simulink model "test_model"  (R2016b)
settings: Solver=VariableStepAuto  StartTime=0.0  StopTime=runtime  RelTol=1e-3
InitFcn:
  | clear mex
  | delete test_model_sfun.mexw64
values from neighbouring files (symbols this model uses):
  g = 9.81    [modelParameters.m]
  height_controlled_o = (((Rm*If        + (((omega0_o * 2 * Rm * Kv * Kq      * Kd + 1)^2) - 1)/(4* Rm*Kv^2*Kq      * Kd))/Vb)*(Pmax - Pmin) + Pmin)    [modelParameters.m]
  If = 0.3836    [modelParameters.m]
  Jreq = 4.2012e-05    [modelParameters.m]
  Jxx = 0.0130    (= 0.013)    [modelParameters.m]
  Jyy = 0.0140    (= 0.014)    [modelParameters.m]
  Jzz = 0.0285    [modelParameters.m]
  Kd = 1.4852e-07    [modelParameters.m]
  Ki_mahony = 0.001    [modelParameters.m]
  Kp_mahony = 0.4    [modelParameters.m]
  Kq = 96.3422    [modelParameters.m]
  Kt = 1.2007e-05    [modelParameters.m]
  Kv = 96.3422    [modelParameters.m]
  m = 1.216    [modelParameters.m]
  omega0_o = sqrt((m*g)/(4*Kt))    [modelParameters.m]
  omega1_o = sqrt((m*g)/(4*Kt))    [modelParameters.m]
  omega2_o = sqrt((m*g)/(4*Kt))    [modelParameters.m]
  omega3_o = sqrt((m*g)/(4*Kt))    [modelParameters.m]
  pitch_o = 0    [modelParameters.m]
  pitchrate_o = 0    [modelParameters.m]
  Pmax = 1    [modelParameters.m]
  Pmin = 0    [modelParameters.m]
  r_oc = [0; 0; 0]    [modelParameters.m]
  rhx = 0.16    [modelParameters.m]
  rhy = 0.16    [modelParameters.m]
  rhz = 0.03    [modelParameters.m]
  Rm = 0.235    [modelParameters.m]
  roll_o = 0    [modelParameters.m]
  rollrate_o = 0    [modelParameters.m]
  Tc = 0.04    [modelParameters.m]
  Tq = 0.005    [modelParameters.m]
  Vb = 11.4    [modelParameters.m]
  x_controlled_o = 0    [modelParameters.m]
  x_o = 0    [modelParameters.m]
  x_vel_o = 0    [modelParameters.m]
  y_controlled_o = 0    [modelParameters.m]
  y_o = 0    [modelParameters.m]
  y_vel_o = 0    [modelParameters.m]
  yaw_controlled_o = 0    [modelParameters.m]
  yaw_o = 0    [modelParameters.m]
  yawrate_o = 0    [modelParameters.m]
  z_o = 0    [modelParameters.m]
  z_vel_o = 0    [modelParameters.m]
undefined symbols (not defined in the file or in its folder): a, Ki, Kp, Ts
libraries: simulink x38, dsparch4 x3, vrlib x2
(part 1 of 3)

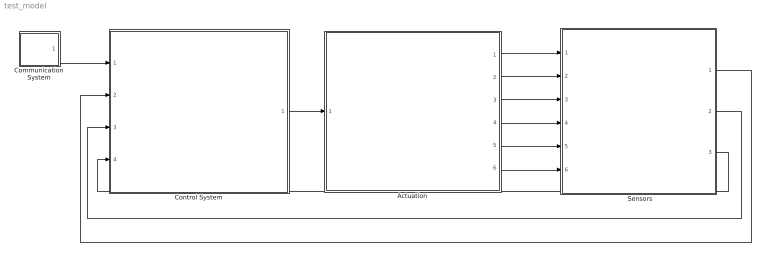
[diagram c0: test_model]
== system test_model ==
  "     Sensors   " : Subsystem
  Actuation : Subsystem
  Communication System : Subsystem
  Control System : Subsystem
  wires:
  Control System/1(P) -> Actuation/1(P)
  Communication System/1(setpoints) -> Control System/1(setpoints)
  Actuation/1(B_omega) -> "     Sensors   "/1(B_Omega)
  Actuation/2(euler_angles) -> "     Sensors   "/2(euler_angles)
  Actuation/3(B_vo) -> "     Sensors   "/3(B_vo)
  Actuation/4(E_ro) -> "     Sensors   "/4(E_ro)
  Actuation/5(B_vo_dot) -> "     Sensors   "/5(B_vo_dot)
  Actuation/6(B_g) -> "     Sensors   "/6(B_g)
  "     Sensors   "/3(current_position) -> Control System/4(current_position)
  "     Sensors   "/2(euler_rates) -> Control System/3(euler_rates)
  "     Sensors   "/1(euler_angles_filtered) -> Control System/2(euler_angles_filtered)

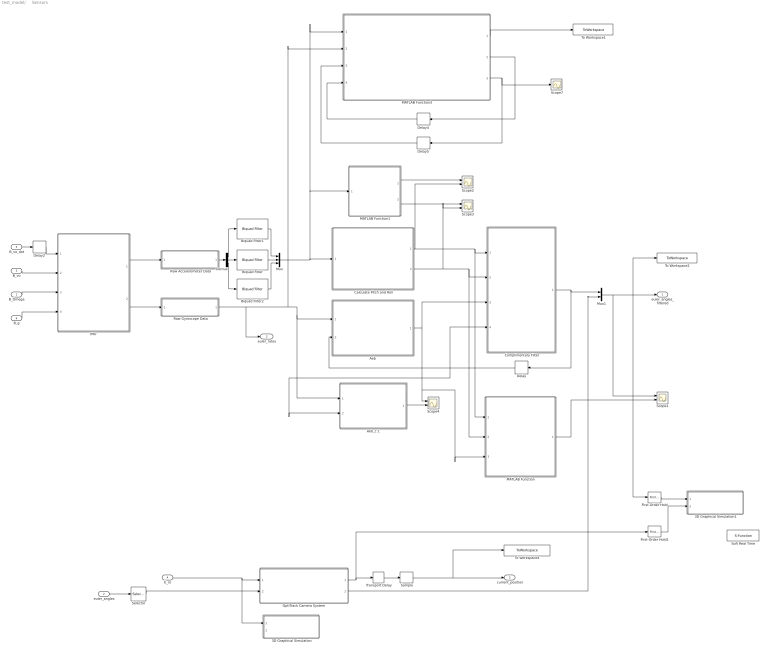
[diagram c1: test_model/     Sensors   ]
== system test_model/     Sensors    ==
  B_Omega : Inport
  euler_angles : Inport  Port=2
  B_vo : Inport  Port=3
  E_ro : Inport  Port=4
  B_vo_dot : Inport  Port=5
  B_g : Inport  Port=6
  3D Graphical Simulation : Subsystem  Commented=on
  3D Graphical Simulation1 : Subsystem  Commented=on
  "Aeb " : MATLAB Function  TreatAsAtomicUnit=on
  Aeb_c 1 : MATLAB Function  TreatAsAtomicUnit=on
  Biquad Filter : dsparch4/Biquad Filter  IIRFiltStruct=Direct form II  CoeffSource=Specify via dialog  BiQuadCoeffs=SOS_Matrix  a0Flag=Warning  IC=0  ICnum=0  ICden=0  InputProcessing=Columns as channels (frame based)  denAccumFracLength=30  denProdOutputFracLength=30  secondMemoryFracLength=15  roundingMode=Floor  overflowMode=off  ScaleValues=1  optimizeScaleValues=on  ScaleValueMode=Specify via input port (g)  scaleValueFracLength=14  FilterSource=Specify via dialog  FilterObject=BQF
  Biquad Filter1 : dsparch4/Biquad Filter  IIRFiltStruct=Direct form II  CoeffSource=Specify via dialog  BiQuadCoeffs=SOS_Matrix  a0Flag=Warning  IC=0  ICnum=0  ICden=0  InputProcessing=Columns as channels (frame based)  denAccumFracLength=30  denProdOutputFracLength=30  secondMemoryFracLength=15  roundingMode=Floor  overflowMode=off  ScaleValues=1  optimizeScaleValues=on  ScaleValueMode=Specify via input port (g)  scaleValueFracLength=14  FilterSource=Specify via dialog  FilterObject=BQF
  Biquad Filter2 : dsparch4/Biquad Filter  IIRFiltStruct=Direct form II  CoeffSource=Specify via dialog  BiQuadCoeffs=SOS_Matrix  a0Flag=Warning  IC=0  ICnum=0  ICden=0  InputProcessing=Columns as channels (frame based)  denAccumFracLength=30  denProdOutputFracLength=30  secondMemoryFracLength=15  roundingMode=Floor  overflowMode=off  ScaleValues=1  optimizeScaleValues=on  ScaleValueMode=Specify via input port (g)  scaleValueFracLength=14  FilterSource=Specify via dialog  FilterObject=BQF
  Calculate Pitch and Roll : MATLAB Function  TreatAsAtomicUnit=on
  Complimentary Filter : MATLAB Function  TreatAsAtomicUnit=on
  Delay : Delay  DelayLength=1  InitialCondition=0
  Delay2 : Delay  DelayLength=1  InitialCondition=0  SampleTime=Tq
  Delay4 : Delay  DelayLength=1  InitialCondition=0  SampleTime=Tq
  Delay5 : Delay  DelayLength=1  InitialCondition=[1, 0, 0, 0]  SampleTime=Tq
  Demux : Demux  Outputs=3
  First-Order Hold : simulink/Discrete/First-Order Hold  DisableCoverage=on  Ts=5e-3
  First-Order Hold1 : simulink/Discrete/First-Order Hold  DisableCoverage=on  Ts=5e-3
  "IMU " : Subsystem
  MATLAB Function : MATLAB Function  TreatAsAtomicUnit=on
  MATLAB Function1 : MATLAB Function  TreatAsAtomicUnit=on
  MATLAB Function3 : MATLAB Function  TreatAsAtomicUnit=on
  Mux : Mux  Inputs=3
  Mux1 : Mux  Inputs=2
  "OptiTrack Camera System " : Subsystem
  Raw Accelerometer Data : Subsystem  Variant=on
  Raw Gyroscope Data : Subsystem  Variant=on
  Sample : ZeroOrderHold  SampleTime=Tc
  Scope{1..4} (4 alike) : Scope  NumInputPorts=2
  Scope7 : Scope
  Selector : Selector  InputPortWidth=3  IndexOptions=Index vector (dialog)  Indices=[3]  OutputSizes=1
  Soft Real Time : S-Function  Commented=on  FunctionName=sfun_time  Parameters=x  SFunctionDeploymentMode=off  EnableBusSupport=off
  To Workspace1 : ToWorkspace  VariableName=mahony_reading  SaveFormat=Structure With Time  SampleTime=Tq
  To Workspace2 : ToWorkspace  VariableName=angle_IMU_reading  SaveFormat=Structure With Time  SampleTime=Tq
  To Workspace4 : ToWorkspace  VariableName=position_model  SaveFormat=Structure With Time  SampleTime=Tc
  Transport Delay : TransportDelay  DelayTime=6e-3
  euler_angles_filtered : Outport
  euler_rates : Outport  Port=2
  current_position : Outport  Port=3
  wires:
  "IMU "/1(accelerometer) -> Raw Accelerometer Data/1(raw_accel_model)
  "IMU "/2(gyroscope) -> Raw Gyroscope Data/1(raw_gyro_model)
  B_vo/1 -> "IMU "/2(B_vo)
  B_Omega/1 -> "IMU "/3(B_Omega)
  B_g/1 -> "IMU "/4(B_g)
  Calculate Pitch and Roll/2(accel_roll) -> Scope3/2, MATLAB Function/2(accel_roll), Complimentary Filter/2(accel_roll)
  Calculate Pitch and Roll/1(accel_pitch) -> MATLAB Function/1(accel_pitch), Complimentary Filter/1(accel_pitch), Scope2/2
  First-Order Hold/1 -> 3D Graphical Simulation1/1("Euler Angles ")
  E_ro/1 -> 3D Graphical Simulation/1(Displacement), "OptiTrack Camera System "/1(E_ro)
  First-Order Hold1/1 -> 3D Graphical Simulation1/2(Displacement)
  B_vo_dot/1 -> Delay2/1
  Delay2/1 -> "IMU "/1(B_vo_dot)
  "OptiTrack Camera System "/1(E_ro_camera) -> Transport Delay/1, First-Order Hold1/1
  Transport Delay/1 -> Sample/1
  Sample/1 -> To Workspace4/1, current_position/1
  Raw Gyroscope Data/1(raw_gyro) -> Aeb_c 1/1(gyro_reading), "Aeb "/1(gyro_reading), MATLAB Function3/2(gyroReadings), euler_rates/1
  Delay/1 -> Complimentary Filter/4(prev_euler_angles), Aeb_c 1/2(euler_angles_filtered), "Aeb "/2(euler_angles_filtered)
  Aeb_c 1/1(euler_rates_IMU) -> Scope4/2
  MATLAB Function1/1(accel_pitch) -> Scope2/1
  MATLAB Function1/2(accel_roll) -> Scope3/1
  "OptiTrack Camera System "/2(yaw_camera) -> Mux1/2
  MATLAB Function3/1(eulerAngles) -> To Workspace1/1
  MATLAB Function3/2(integralFeedback) -> Delay4/1
  Delay4/1 -> MATLAB Function3/4(integralFeedback_prev)
  MATLAB Function3/3(quaternions) -> Scope7/1, Delay5/1
  Delay5/1 -> MATLAB Function3/3(quaternions_prev)
  "Aeb "/1(euler_rates_IMU) -> MATLAB Function/3(euler_rates_gyro), Scope4/1, Complimentary Filter/3(euler_rates_gyro)
  Raw Accelerometer Data/1(raw_accel) -> Demux/1
  Demux/2 -> Biquad Filter/1
  Demux/1 -> Biquad Filter1/1
  Demux/3 -> Biquad Filter2/1
  Biquad Filter/1 -> Mux/2
  Biquad Filter1/1 -> Mux/1
  Biquad Filter2/1 -> Mux/3
  Mux/1 -> Calculate Pitch and Roll/1(accel_reading), MATLAB Function1/1(accel_reading), MATLAB Function3/1(accelReadings)
  Complimentary Filter/1(euler_angles_IMU) -> Mux1/1, Delay/1
  euler_angles/1 -> Selector/1
  Selector/1 -> "OptiTrack Camera System "/2(yaw)
  MATLAB Function/1(euler_angles_IMU) -> Scope1/2
  Mux1/1 -> Scope1/1, To Workspace2/1, First-Order Hold/1, euler_angles_filtered/1

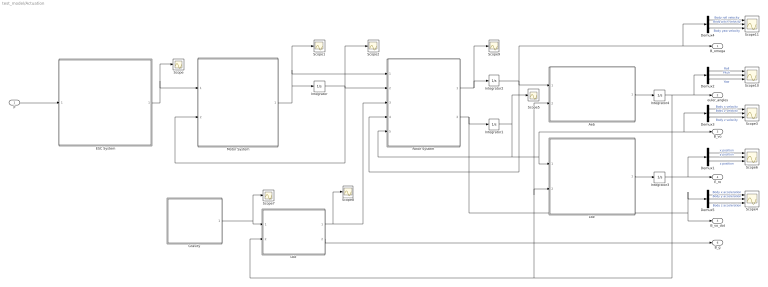
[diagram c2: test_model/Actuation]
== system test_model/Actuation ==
  P : Inport
  "Aeb " : MATLAB Function  TreatAsAtomicUnit=on
  Demux{1..5} (5 alike) : Demux  Outputs=3
  ESC System : MATLAB Function  TreatAsAtomicUnit=on
  "Gravity " : MATLAB Function  TreatAsAtomicUnit=on
  Integrator : Integrator  InitialCondition=[omega0_o, omega1_o, omega2_o, omega3_o]
  Integrator1 : Integrator  InitialCondition=[x_vel_o; y_vel_o; z_vel_o]
  Integrator2 : Integrator  InitialCondition=[rollrate_o; pitchrate_o; yawrate_o]
  Integrator3 : Integrator  InitialCondition=[x_o; y_o; z_o]
  Integrator4 : Integrator  InitialCondition=[roll_o; pitch_o; yaw_o]  ContinuousStateAttributes=['phi' 'theta' 'psi']
  "Lbe " : MATLAB Function  TreatAsAtomicUnit=on
  "Lbe " : MATLAB Function  TreatAsAtomicUnit=on
  Motor System : MATLAB Function  TreatAsAtomicUnit=on
  "Rotor System " : MATLAB Function  TreatAsAtomicUnit=on
  Scope{,1..2,5,7..9} (7 alike) : Scope
  Scope{3..4,6,10..11} (5 alike) : Scope  NumInputPorts=3
  B_omega : Outport
  euler_angles : Outport  Port=2
  B_vo : Outport  Port=3
  E_ro : Outport  Port=4
  B_vo_dot : Outport  Port=5
  B_g : Outport  Port=6
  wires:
  ESC System/1(Vb_eff) -> Scope/1, Motor System/1(Vb_eff)
  Motor System/1(w_dot) -> Integrator/1, Scope1/1, "Rotor System "/1(w_dot)
  "Rotor System "/1(B_omega_dot) -> Scope9/1, Integrator2/1
  Integrator2/1 -> "Rotor System "/4(B_omega), B_omega/1, Demux4/1, "Aeb "/1(B_omega)
  "Aeb "/1(euler_rates) -> Integrator4/1
  "Lbe "/1(E_ro) -> Integrator3/1
  Integrator3/1 -> Demux1/1, E_ro/1
  "Lbe "/1(B_Fg) -> Scope8/1, "Rotor System "/3(B_Fg)
  "Lbe "/2(B_g) -> B_g/1
  Demux1/2 -> Scope6/2  "y position"
  Demux1/1 -> Scope6/1  "x position"
  Demux1/3 -> Scope6/3  "z position"
  Demux2/2 -> Scope10/2  "Pitch"
  Demux2/1 -> Scope10/1  "Roll"
  Demux2/3 -> Scope10/3  "Yaw"
  Demux4/2 -> Scope11/2  "Body pitch velocity"
  Demux4/1 -> Scope11/1  "Body roll velocity"
  Demux4/3 -> Scope11/3  "Body yaw velocity"
  Demux3/2 -> Scope3/2  "Body y velocity"
  Demux3/1 -> Scope3/1  "Body x velocity"
  Demux3/3 -> Scope3/3  "Body z velocity"
  Demux5/2 -> Scope4/2  "Body y acceleration"
  Demux5/1 -> Scope4/1  "Body x acceleration"
  Demux5/3 -> Scope4/3  "Body z acceleration"
  Integrator1/1 -> Scope5/1, "Rotor System "/5(B_vo), "Lbe "/1(B_vo), Demux3/1, B_vo/1
  "Rotor System "/2(B_vo_dot) -> Demux5/1, B_vo_dot/1, Integrator1/1
  Integrator4/1 -> euler_angles/1, Demux2/1, "Lbe "/2(euler_angles), "Aeb "/2(euler_angles), "Lbe "/2(euler_angles)
  P/1 -> ESC System/1(P)
  "Gravity "/1(E_Fg) -> Scope7/1, "Lbe "/1(E_Fg)
  Integrator/1 -> Motor System/2(w), "Rotor System "/2(w), Scope2/1

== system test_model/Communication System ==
  Step : Step  Before=[0; 0; 0; 0]  After=[0; 1; 0; 0]  SampleTime=Tq
  setpoints : Outport
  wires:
  Step/1 -> setpoints/1

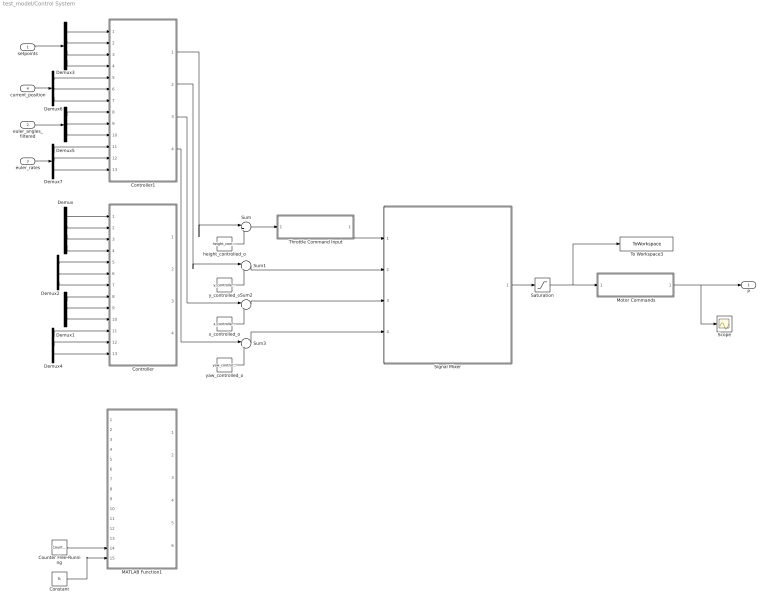
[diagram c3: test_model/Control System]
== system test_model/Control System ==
  setpoints : Inport
  euler_angles_filtered : Inport  Port=2
  euler_rates : Inport  Port=3
  current_position : Inport  Port=4
  Constant : Constant  Value=Tc  SampleTime=Tc
  Controller : Subsystem  Commented=on
  Controller1 : Subsystem
  Counter Free-Running : simulink/Sources/Counter Free-Running  NumBits=32  tsamp=Tc
  Demux : Demux
  Demux{1..2,4..7} (6 alike) : Demux  Outputs=3
  Demux3 : Demux
  MATLAB Function1 : MATLAB Function  Commented=on  TreatAsAtomicUnit=on  SystemSampleTime=Tq
  Motor Commands : Subsystem  Variant=on
  Saturation : Saturate  UpperLimit=Pmax*ones(4,1)  LowerLimit=Pmin*ones(4,1)
  Scope : Scope
  Signal Mixer : MATLAB Function  TreatAsAtomicUnit=on
  Sum{,1..3} (4 alike) : Sum  Inputs=|++
  Throttle Command Input : Subsystem  Variant=on
  To Workspace3 : ToWorkspace  VariableName=motorCommands  SaveFormat=Structure With Time  SampleTime=Tq
  height_controlled_o : Constant  Value=height_controlled_o  SampleTime=Tc
  x_controlled_o : Constant  Value=x_controlled_o
  y_controlled_o : Constant  Value=y_controlled_o
  yaw_controlled_o : Constant  Value=yaw_controlled_o
  P : Outport
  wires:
  Demux/1 -> Controller/1(x_setpoint)
  Demux/2 -> Controller/2(y_setpoint)
  Demux/3 -> Controller/3(z_setpoint)
  Demux2/1 -> Controller/5(x_position)
  Demux2/2 -> Controller/6(y_position)
  Demux2/3 -> Controller/7(z_position)
  y_controlled_o/1 -> Sum1/2
  x_controlled_o/1 -> Sum2/2
  yaw_controlled_o/1 -> Sum3/2
  Signal Mixer/1(P) -> Saturation/1
  Demux1/1 -> Controller/8(roll)
  Demux1/2 -> Controller/9(pitch)
  Demux4/1 -> Controller/11(roll_rate)
  Demux4/2 -> Controller/12(pitch_rate)
  Demux4/3 -> Controller/13(yaw_rate)
  Demux/4 -> Controller/4(yaw_setpoint)
  Demux1/3 -> Controller/10(yaw)
  Counter Free-Running/1 -> MATLAB Function1/14(vrpn_id)
  Constant/1 -> MATLAB Function1/15(Tc)
  Sum1/1 -> Signal Mixer/2(y_controlled)
  Sum2/1 -> Signal Mixer/3(x_controlled)
  Sum3/1 -> Signal Mixer/4(yaw_controlled)
  Throttle Command Input/1(z_command) -> Signal Mixer/1(height_controlled)
  height_controlled_o/1 -> Sum/2
  Motor Commands/1(z_command) -> P/1, Scope/1
  Sum/1 -> Throttle Command Input/1(z_command_model)
  Saturation/1 -> To Workspace3/1, Motor Commands/1(z_command_model)
  setpoints/1 -> Demux3/1
  current_position/1 -> Demux6/1
  euler_angles_filtered/1 -> Demux5/1
  euler_rates/1 -> Demux7/1
  Demux3/1 -> Controller1/1(x_setpoint)
  Demux3/2 -> Controller1/2(y_setpoint)
  Demux3/3 -> Controller1/3(z_setpoint)
  Demux3/4 -> Controller1/4(yaw_setpoint)
  Demux6/1 -> Controller1/5(x_position)
  Demux6/2 -> Controller1/6(y_position)
  Demux6/3 -> Controller1/7(z_position)
  Demux5/1 -> Controller1/8(roll)
  Demux5/2 -> Controller1/9(pitch)
  Demux5/3 -> Controller1/10(yaw)
  Demux7/1 -> Controller1/11(roll_rate)
  Demux7/2 -> Controller1/12(pitch_rate)
  Demux7/3 -> Controller1/13(yaw_rate)
  Controller1/4(yaw_controlled) -> Sum3/1
  Controller1/3(x_controlled) -> Sum2/1
  Controller1/2(y_controlled) -> Sum1/1
  Controller1/1(height_controlled) -> Sum/1

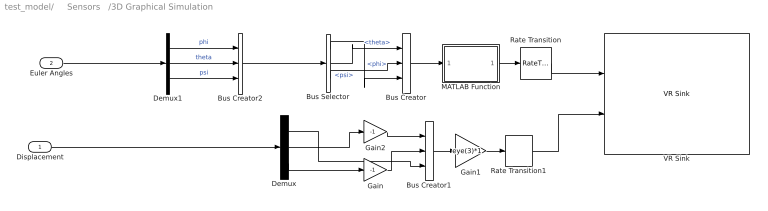
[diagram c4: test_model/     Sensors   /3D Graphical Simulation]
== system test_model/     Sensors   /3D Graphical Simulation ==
  Displacement : Inport
  Euler Angles : Inport  Port=2
  Bus Creator : BusCreator  Inputs=3
  Bus Creator1 : BusCreator  Inputs=3
  Bus Creator2 : BusCreator  Inputs=3
  Bus Selector : BusSelector  OutputSignals=phi,theta,psi
  Demux : Demux  Outputs=3
  Demux1 : Demux  Outputs=3
  Gain : Gain  Gain=-1
  Gain1 : Gain  Gain=eye(3)*1  Multiplication=Matrix(K*u)
  Gain2 : Gain  Gain=-1
  MATLAB Function : MATLAB Function  TreatAsAtomicUnit=on
  Rate Transition : RateTransition  OutPortSampleTime=0.06
  Rate Transition1 : RateTransition  OutPortSampleTime=0.06
  VR Sink : vrlib/VR Sink  InstantiateOnLoad=on  SampleTime=-1  ViewEnable=on  RemoteChange=off  RemoteView=off  FieldsWritten=Helicopter.rotation.4.1.1.double#Helicopter.translation.3.1.1.double  WorldFileName=quadrotor_world_ucart.wrl  AutoView=on  VideoDimensions=[]  AllowVariableSize=off
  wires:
  Displacement/1 -> Demux/1
  Bus Creator2/1 -> Bus Selector/1
  Demux/1 -> Bus Creator1/3
  Gain/1 -> Bus Creator1/2
  Gain2/1 -> Bus Creator1/1
  Rate Transition1/1 -> VR Sink/2
  Rate Transition/1 -> VR Sink/1
  Demux/3 -> Gain/1
  Demux/2 -> Gain2/1
  Bus Creator1/1 -> Gain1/1
  Bus Selector/1 -> Bus Creator/3  "<phi>"
  Bus Selector/3 -> Bus Creator/2  "<psi>"
  Bus Selector/2 -> Bus Creator/1  "<theta>"
  Gain1/1 -> Rate Transition1/1
  Demux1/3 -> Bus Creator2/3  "psi"
  Demux1/2 -> Bus Creator2/2  "theta"
  Demux1/1 -> Bus Creator2/1  "phi"
  Euler Angles/1 -> Demux1/1
  Bus Creator/1 -> MATLAB Function/1(u)
  MATLAB Function/1(y) -> Rate Transition/1

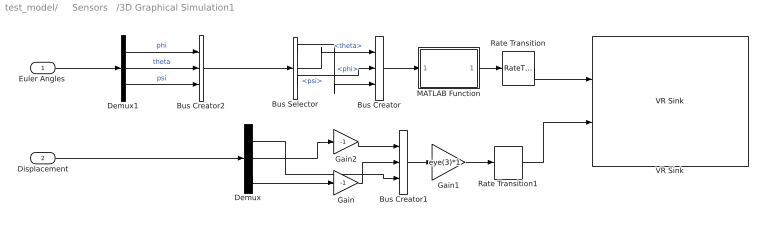
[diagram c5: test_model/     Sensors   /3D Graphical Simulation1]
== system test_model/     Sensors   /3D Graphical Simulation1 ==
  "Euler Angles " : Inport
  Displacement : Inport  Port=2
  Bus Creator : BusCreator  Inputs=3
  Bus Creator1 : BusCreator  Inputs=3
  Bus Creator2 : BusCreator  Inputs=3
  Bus Selector : BusSelector  OutputSignals=phi,theta,psi
  Demux : Demux  Outputs=3
  Demux1 : Demux  Outputs=3
  Gain : Gain  Gain=-1
  Gain1 : Gain  Gain=eye(3)*1  Multiplication=Matrix(K*u)
  Gain2 : Gain  Gain=-1
  MATLAB Function : MATLAB Function  TreatAsAtomicUnit=on
  Rate Transition : RateTransition  OutPortSampleTime=0.06
  Rate Transition1 : RateTransition  OutPortSampleTime=0.06
  VR Sink : vrlib/VR Sink  InstantiateOnLoad=on  SampleTime=-1  ViewEnable=on  RemoteChange=off  RemoteView=off  FieldsWritten=Helicopter.rotation.4.1.1.double#Helicopter.translation.3.1.1.double  WorldFileName=quadrotor_world_ucart.wrl  AutoView=on  VideoDimensions=[]  AllowVariableSize=off
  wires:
  Bus Creator2/1 -> Bus Selector/1
  Demux/1 -> Bus Creator1/3
  Gain/1 -> Bus Creator1/2
  Gain2/1 -> Bus Creator1/1
  Rate Transition1/1 -> VR Sink/2
  Rate Transition/1 -> VR Sink/1
  Demux/3 -> Gain/1
  Demux/2 -> Gain2/1
  Bus Creator1/1 -> Gain1/1
  Bus Selector/1 -> Bus Creator/3  "<phi>"
  Bus Selector/3 -> Bus Creator/2  "<psi>"
  Bus Selector/2 -> Bus Creator/1  "<theta>"
  Gain1/1 -> Rate Transition1/1
  Demux1/3 -> Bus Creator2/3  "psi"
  Demux1/2 -> Bus Creator2/2  "theta"
  Demux1/1 -> Bus Creator2/1  "phi"
  Bus Creator/1 -> MATLAB Function/1(u)
  MATLAB Function/1(y) -> Rate Transition/1
  Displacement/1 -> Demux/1
  "Euler Angles "/1 -> Demux1/1

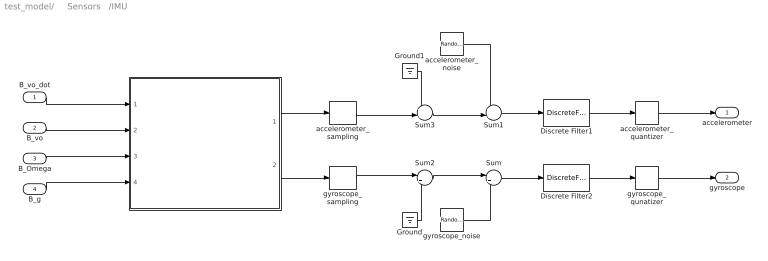
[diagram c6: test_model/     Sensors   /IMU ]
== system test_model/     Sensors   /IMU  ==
  B_vo_dot : Inport
  B_vo : Inport  Port=2
  B_Omega : Inport  Port=3
  B_g : Inport  Port=4
  " " : MATLAB Function  TreatAsAtomicUnit=on
  Discrete Filter1 : DiscreteFilter  Numerator=[0 0.749]  Denominator=[1 -0.251]  InitialStates=[0, 0, -1]  SampleTime=Tq
  Discrete Filter2 : DiscreteFilter  Numerator=[0 0.7327]  Denominator=[1 -0.2673]  SampleTime=Tq
  Ground : Ground
  Ground1 : Ground
  Sum : Sum  Inputs=|++
  Sum1 : Sum  Inputs=++|
  Sum2 : Sum  Inputs=|++
  Sum3 : Sum  Inputs=++|
  accelerometer_noise : RandomNumber  Mean=zeros(3,1)  Variance=[ 3e-7 ; 3.3e-7 ; 7.2e-7 ]  Seed=[0,1,2]  SampleTime=Tq
  accelerometer_quantizer : Quantizer  QuantizationInterval=2.4400e-04
  accelerometer_sampling : ZeroOrderHold  SampleTime=Tq
  gyroscope_noise : RandomNumber  Mean=zeros(3,1)  Variance=[ 2.2e-8 ; 1.1e-7 ; 2.4e-8 ]  Seed=[0,1,2]  SampleTime=Tq
  gyroscope_qunatizer : Quantizer  QuantizationInterval=1.1e-3
  gyroscope_sampling : ZeroOrderHold  SampleTime=Tq
  accelerometer : Outport
  gyroscope : Outport  Port=2
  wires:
  accelerometer_noise/1 -> Sum1/1
  Sum2/1 -> Sum/1
  Sum3/1 -> Sum1/2
  gyroscope_noise/1 -> Sum/2
  gyroscope_sampling/1 -> Sum2/1
  accelerometer_sampling/1 -> Sum3/2
  Ground/1 -> Sum2/2
  Ground1/1 -> Sum3/1
  B_vo_dot/1 -> " "/1(B_vo_dot)
  B_vo/1 -> " "/2(B_vo)
  B_Omega/1 -> " "/3(B_Omega)
  B_g/1 -> " "/4(B_g)
  " "/2(gyroReading) -> gyroscope_sampling/1
  " "/1(accelReading) -> accelerometer_sampling/1
  Sum1/1 -> Discrete Filter1/1
  Sum/1 -> Discrete Filter2/1
  accelerometer_quantizer/1 -> accelerometer/1
  gyroscope_qunatizer/1 -> gyroscope/1
  Discrete Filter1/1 -> accelerometer_quantizer/1
  Discrete Filter2/1 -> gyroscope_qunatizer/1

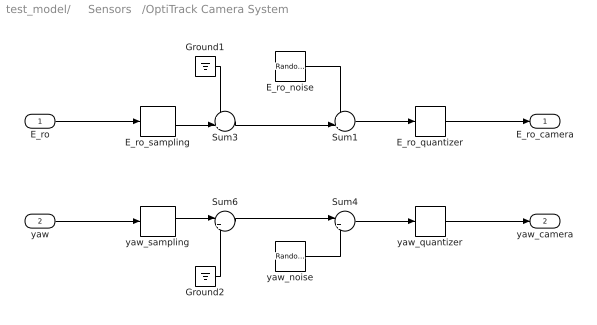
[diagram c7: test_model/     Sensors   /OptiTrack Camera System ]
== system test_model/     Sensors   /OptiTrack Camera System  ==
  E_ro : Inport
  yaw : Inport  Port=2
  E_ro_noise : RandomNumber  Mean=zeros(3,1)  Variance=[ 7.9664e-10 ; 1.1928e-10 ; 5.0636e-10 ]  Seed=[0,1,2]  SampleTime=Tc
  E_ro_quantizer : Quantizer  QuantizationInterval=2.4400e-04
  E_ro_sampling : ZeroOrderHold  SampleTime=Tc
  Ground1 : Ground
  Ground2 : Ground
  Sum1 : Sum  Inputs=++|
  Sum3 : Sum  Inputs=++|
  Sum4 : Sum  Inputs=|++
  Sum6 : Sum  Inputs=|++
  yaw_noise : RandomNumber  Variance=1.0783e-9  SampleTime=Tq
  yaw_quantizer : Quantizer  QuantizationInterval=1.1e-3
  yaw_sampling : ZeroOrderHold  SampleTime=Tq
  E_ro_camera : Outport
  yaw_camera : Outport  Port=2
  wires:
  E_ro_noise/1 -> Sum1/1
  Sum3/1 -> Sum1/2
  Sum1/1 -> E_ro_quantizer/1
  E_ro_sampling/1 -> Sum3/2
  Ground1/1 -> Sum3/1
  Sum4/1 -> yaw_quantizer/1
  Sum6/1 -> Sum4/1
  yaw_noise/1 -> Sum4/2
  yaw_sampling/1 -> Sum6/1
  Ground2/1 -> Sum6/2
  yaw/1 -> yaw_sampling/1
  E_ro/1 -> E_ro_sampling/1
  E_ro_quantizer/1 -> E_ro_camera/1
  yaw_quantizer/1 -> yaw_camera/1

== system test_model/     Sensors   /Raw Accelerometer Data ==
  note: 1) Add Subsystem or Model blocks as valid variant choices. 2) You cannot connect blocks at this level. At simulation, connectivity is automatically determined, based on the active variant and port name matching.
  raw_accel_model : Inport
  Feedback : Subsystem  VariantControl=logAnalysisToggle==0
  "Raw Accelerometer Data " : Subsystem  VariantControl=logAnalysisToggle==1
  raw_accel : Outport

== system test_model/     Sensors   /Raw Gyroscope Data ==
  note: 1) Add Subsystem or Model blocks as valid variant choices. 2) You cannot connect blocks at this level. At simulation, connectivity is automatically determined, based on the active variant and port name matching.
  raw_gyro_model : Inport
  Feedback : Subsystem  VariantControl=logAnalysisToggle==0
  "Raw Gyroscope Data " : Subsystem  VariantControl=logAnalysisToggle==1
  raw_gyro : Outport

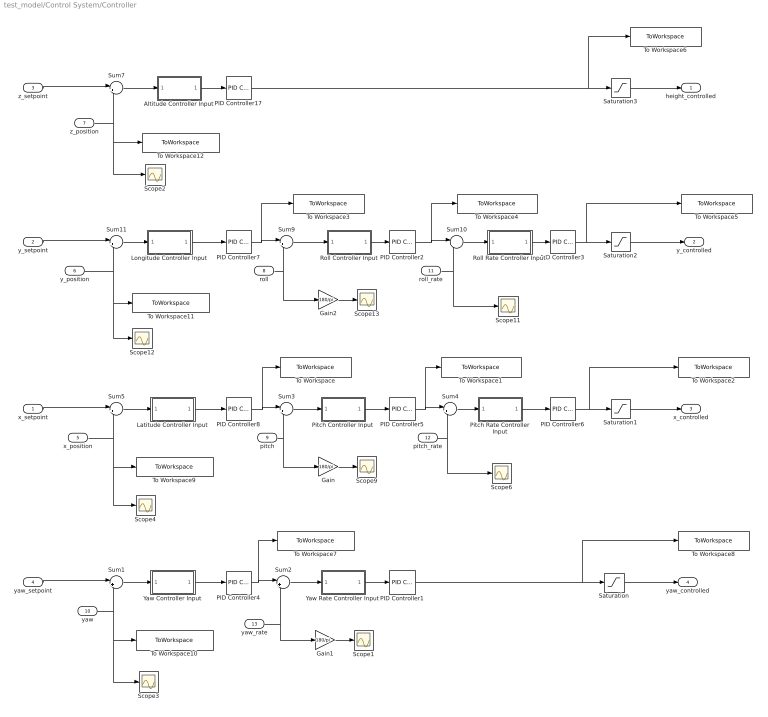
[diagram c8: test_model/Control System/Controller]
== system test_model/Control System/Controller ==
  x_setpoint : Inport
  y_setpoint : Inport  Port=2
  z_setpoint : Inport  Port=3
  yaw_setpoint : Inport  Port=4
  x_position : Inport  Port=5
  y_position : Inport  Port=6
  z_position : Inport  Port=7
  roll : Inport  Port=8
  pitch : Inport  Port=9
  yaw : Inport  Port=10
  roll_rate : Inport  Port=11
  pitch_rate : Inport  Port=12
  yaw_rate : Inport  Port=13
  Altitude Controller Input : Subsystem  Variant=on
  Gain : Gain  Gain=180/pi
  Gain1 : Gain  Gain=180/pi
  Gain2 : Gain  Gain=180/pi
  Latitude Controller Input : Subsystem  Variant=on
  Longitude Controller Input : Subsystem  Variant=on
  PID Controller1 : simulink/Continuous/PID Controller  Controller=P  TimeDomain=Discrete-time  SampleTime=Tq  IntegratorMethod=Forward Euler  FilterMethod=Forward Euler  Form=Parallel  UseFilter=on  ControllerParametersSource=internal  P=29700  I=-77.7  D=2.32  N=1/0.0818  InitialConditionSource=internal  InitialConditionForIntegrator=0  InitialConditionForFilter=0  ExternalReset=none  ZeroCross=off  LimitOutput=off  UpperSaturationLimit=inf  LowerSaturationLimit=-inf  LinearizeAsGain=on  AntiWindupMode=none  Kb=1  TrackingMode=off  Kt=1  PParamMin=[]  PParamMax=[]  IParamMin=[]  IParamMax=[]  DParamMin=[]  DParamMax=[]  NParamMin=[]  NParamMax=[]  KbParamMin=[]  KbParamMax=[]  KtParamMin=[]  KtParamMax=[]  POutMin=[]  POutMax=[]  IOutMin=[]  IOutMax=[]  DOutMin=[]  DOutMax=[]  NOutMin=[]  NOutMax=[]  KbOutMin=[]  KbOutMax=[]  KtOutMin=[]  KtOutMax=[]  IntegratorOutMin=[]  IntegratorOutMax=[]  FilterOutMin=[]  FilterOutMax=[]  SumOutMin=[]  SumOutMax=[]  SumI1OutMin=[]  SumI1OutMax=[]  SumI2OutMin=[]  SumI2OutMax=[]  SumI3OutMin=[]  SumI3OutMax=[]  SumDOutMin=[]  SumDOutMax=[]  SaturationOutMin=[]  SaturationOutMax=[]  IntegratorContinuousStateAttributes=''  IntegratorStateMustResolveToSignalObject=off  IntegratorRTWStateStorageClass=Auto  FilterContinuousStateAttributes=''  FilterStateMustResolveToSignalObject=off  FilterRTWStateStorageClass=Auto  DifferentiatorICPrevScaledInput=0  DifferentiatorOutMin=[]  DifferentiatorOutMax=[]
  PID Controller17 : simulink/Continuous/PID Controller  Controller=PID  TimeDomain=Discrete-time  SampleTime=Tc  IntegratorMethod=Forward Euler  FilterMethod=Forward Euler  Form=Parallel  UseFilter=on  ControllerParametersSource=internal  P=-9804  I=-817  D=-7353  N=3  InitialConditionSource=internal  InitialConditionForIntegrator=0  InitialConditionForFilter=0  ExternalReset=none  LimitOutput=off  UpperSaturationLimit=inf  LowerSaturationLimit=-inf  LinearizeAsGain=on  AntiWindupMode=none  Kb=1  TrackingMode=off  Kt=1  PParamMin=[]  PParamMax=[]  IParamMin=[]  IParamMax=[]  DParamMin=[]  DParamMax=[]  NParamMin=[]  NParamMax=[]  KbParamMin=[]  KbParamMax=[]  KtParamMin=[]  KtParamMax=[]  POutMin=[]  POutMax=[]  IOutMin=[]  IOutMax=[]  DOutMin=[]  DOutMax=[]  NOutMin=[]  NOutMax=[]  KbOutMin=[]  KbOutMax=[]  KtOutMin=[]  KtOutMax=[]  IntegratorOutMin=[]  IntegratorOutMax=[]  FilterOutMin=[]  FilterOutMax=[]  SumOutMin=[]  SumOutMax=[]  SumI1OutMin=[]  SumI1OutMax=[]  SumI2OutMin=[]  SumI2OutMax=[]  SumI3OutMin=[]  SumI3OutMax=[]  SumDOutMin=[]  SumDOutMax=[]  SaturationOutMin=[]  SaturationOutMax=[]  IntegratorContinuousStateAttributes=''  IntegratorStateMustResolveToSignalObject=off  IntegratorRTWStateStorageClass=Auto  FilterContinuousStateAttributes=''  FilterStateMustResolveToSignalObject=off  FilterRTWStateStorageClass=Auto  DifferentiatorICPrevScaledInput=0  DifferentiatorOutMin=[]  DifferentiatorOutMax=[]
  PID Controller2 : simulink/Continuous/PID Controller  Controller=PD  TimeDomain=Discrete-time  SampleTime=Tq  IntegratorMethod=Forward Euler  FilterMethod=Forward Euler  Form=Parallel  UseFilter=off  ControllerParametersSource=internal  P=15  I=35.1207902652377  D=0.2  N=3  InitialConditionSource=internal  InitialConditionForIntegrator=0  InitialConditionForFilter=0  ExternalReset=none  LimitOutput=off  UpperSaturationLimit=inf  LowerSaturationLimit=-inf  LinearizeAsGain=on  AntiWindupMode=none  Kb=1  TrackingMode=off  Kt=1  PParamMin=[]  PParamMax=[]  IParamMin=[]  IParamMax=[]  DParamMin=[]  DParamMax=[]  NParamMin=[]  NParamMax=[]  KbParamMin=[]  KbParamMax=[]  KtParamMin=[]  KtParamMax=[]  POutMin=[]  POutMax=[]  IOutMin=[]  IOutMax=[]  DOutMin=[]  DOutMax=[]  NOutMin=[]  NOutMax=[]  KbOutMin=[]  KbOutMax=[]  KtOutMin=[]  KtOutMax=[]  IntegratorOutMin=[]  IntegratorOutMax=[]  FilterOutMin=[]  FilterOutMax=[]  SumOutMin=[]  SumOutMax=[]  SumI1OutMin=[]  SumI1OutMax=[]  SumI2OutMin=[]  SumI2OutMax=[]  SumI3OutMin=[]  SumI3OutMax=[]  SumDOutMin=[]  SumDOutMax=[]  SaturationOutMin=[]  SaturationOutMax=[]  IntegratorContinuousStateAttributes=''  IntegratorStateMustResolveToSignalObject=off  IntegratorRTWStateStorageClass=Auto  FilterContinuousStateAttributes=''  FilterStateMustResolveToSignalObject=off  FilterRTWStateStorageClass=Auto  DifferentiatorICPrevScaledInput=0  DifferentiatorOutMin=[]  DifferentiatorOutMax=[]
  PID Controller3 : simulink/Continuous/PID Controller  Controller=PD  TimeDomain=Discrete-time  SampleTime=Tq  IntegratorMethod=Forward Euler  FilterMethod=Forward Euler  Form=Parallel  UseFilter=off  ControllerParametersSource=internal  P=4600  I=1575.82088970639  D=550  N=3  InitialConditionSource=internal  InitialConditionForIntegrator=0  InitialConditionForFilter=0  ExternalReset=none  LimitOutput=off  UpperSaturationLimit=inf  LowerSaturationLimit=-inf  LinearizeAsGain=on  AntiWindupMode=none  Kb=1  TrackingMode=off  Kt=1  PParamMin=[]  PParamMax=[]  IParamMin=[]  IParamMax=[]  DParamMin=[]  DParamMax=[]  NParamMin=[]  NParamMax=[]  KbParamMin=[]  KbParamMax=[]  KtParamMin=[]  KtParamMax=[]  POutMin=[]  POutMax=[]  IOutMin=[]  IOutMax=[]  DOutMin=[]  DOutMax=[]  NOutMin=[]  NOutMax=[]  KbOutMin=[]  KbOutMax=[]  KtOutMin=[]  KtOutMax=[]  IntegratorOutMin=[]  IntegratorOutMax=[]  FilterOutMin=[]  FilterOutMax=[]  SumOutMin=[]  SumOutMax=[]  SumI1OutMin=[]  SumI1OutMax=[]  SumI2OutMin=[]  SumI2OutMax=[]  SumI3OutMin=[]  SumI3OutMax=[]  SumDOutMin=[]  SumDOutMax=[]  SaturationOutMin=[]  SaturationOutMax=[]  IntegratorContinuousStateAttributes=''  IntegratorStateMustResolveToSignalObject=off  IntegratorRTWStateStorageClass=Auto  FilterContinuousStateAttributes=''  FilterStateMustResolveToSignalObject=off  FilterRTWStateStorageClass=Auto  DifferentiatorICPrevScaledInput=0  DifferentiatorOutMin=[]  DifferentiatorOutMax=[]
  PID Controller4 : simulink/Continuous/PID Controller  Controller=PD  TimeDomain=Discrete-time  SampleTime=Tc  IntegratorMethod=Forward Euler  FilterMethod=Forward Euler  Form=Parallel  UseFilter=off  ControllerParametersSource=internal  P=2.6  I=2.36803176515497  D=0  N=3.83298618768959  InitialConditionSource=internal  InitialConditionForIntegrator=0  InitialConditionForFilter=0  ExternalReset=none  LimitOutput=off  UpperSaturationLimit=inf  LowerSaturationLimit=-inf  LinearizeAsGain=on  AntiWindupMode=none  Kb=1  TrackingMode=off  Kt=1  PParamMin=[]  PParamMax=[]  IParamMin=[]  IParamMax=[]  DParamMin=[]  DParamMax=[]  NParamMin=[]  NParamMax=[]  KbParamMin=[]  KbParamMax=[]  KtParamMin=[]  KtParamMax=[]  POutMin=[]  POutMax=[]  IOutMin=[]  IOutMax=[]  DOutMin=[]  DOutMax=[]  NOutMin=[]  NOutMax=[]  KbOutMin=[]  KbOutMax=[]  KtOutMin=[]  KtOutMax=[]  IntegratorOutMin=[]  IntegratorOutMax=[]  FilterOutMin=[]  FilterOutMax=[]  SumOutMin=[]  SumOutMax=[]  SumI1OutMin=[]  SumI1OutMax=[]  SumI2OutMin=[]  SumI2OutMax=[]  SumI3OutMin=[]  SumI3OutMax=[]  SumDOutMin=[]  SumDOutMax=[]  SaturationOutMin=[]  SaturationOutMax=[]  IntegratorContinuousStateAttributes=''  IntegratorStateMustResolveToSignalObject=off  IntegratorRTWStateStorageClass=Auto  FilterContinuousStateAttributes=''  FilterStateMustResolveToSignalObject=off  FilterRTWStateStorageClass=Auto  DifferentiatorICPrevScaledInput=0  DifferentiatorOutMin=[]  DifferentiatorOutMax=[]
  PID Controller5 : simulink/Continuous/PID Controller  Controller=PD  TimeDomain=Discrete-time  SampleTime=Tq  IntegratorMethod=Forward Euler  FilterMethod=Forward Euler  Form=Parallel  UseFilter=off  ControllerParametersSource=internal  P=15  I=35.1207902652377  D=0.2  N=3  InitialConditionSource=internal  InitialConditionForIntegrator=0  InitialConditionForFilter=0  ExternalReset=none  LimitOutput=off  UpperSaturationLimit=inf  LowerSaturationLimit=-inf  LinearizeAsGain=on  AntiWindupMode=none  Kb=1  TrackingMode=off  Kt=1  PParamMin=[]  PParamMax=[]  IParamMin=[]  IParamMax=[]  DParamMin=[]  DParamMax=[]  NParamMin=[]  NParamMax=[]  KbParamMin=[]  KbParamMax=[]  KtParamMin=[]  KtParamMax=[]  POutMin=[]  POutMax=[]  IOutMin=[]  IOutMax=[]  DOutMin=[]  DOutMax=[]  NOutMin=[]  NOutMax=[]  KbOutMin=[]  KbOutMax=[]  KtOutMin=[]  KtOutMax=[]  IntegratorOutMin=[]  IntegratorOutMax=[]  FilterOutMin=[]  FilterOutMax=[]  SumOutMin=[]  SumOutMax=[]  SumI1OutMin=[]  SumI1OutMax=[]  SumI2OutMin=[]  SumI2OutMax=[]  SumI3OutMin=[]  SumI3OutMax=[]  SumDOutMin=[]  SumDOutMax=[]  SaturationOutMin=[]  SaturationOutMax=[]  IntegratorContinuousStateAttributes=''  IntegratorStateMustResolveToSignalObject=off  IntegratorRTWStateStorageClass=Auto  FilterContinuousStateAttributes=''  FilterStateMustResolveToSignalObject=off  FilterRTWStateStorageClass=Auto  DifferentiatorICPrevScaledInput=0  DifferentiatorOutMin=[]  DifferentiatorOutMax=[]
  PID Controller6 : simulink/Continuous/PID Controller  Controller=PD  TimeDomain=Discrete-time  SampleTime=Tq  IntegratorMethod=Forward Euler  FilterMethod=Forward Euler  Form=Parallel  UseFilter=off  ControllerParametersSource=internal  P=4600  I=1575.82088970639  D=550  N=3  InitialConditionSource=internal  InitialConditionForIntegrator=0  InitialConditionForFilter=0  ExternalReset=none  LimitOutput=off  UpperSaturationLimit=inf  LowerSaturationLimit=-inf  LinearizeAsGain=on  AntiWindupMode=none  Kb=1  TrackingMode=off  Kt=1  PParamMin=[]  PParamMax=[]  IParamMin=[]  IParamMax=[]  DParamMin=[]  DParamMax=[]  NParamMin=[]  NParamMax=[]  KbParamMin=[]  KbParamMax=[]  KtParamMin=[]  KtParamMax=[]  POutMin=[]  POutMax=[]  IOutMin=[]  IOutMax=[]  DOutMin=[]  DOutMax=[]  NOutMin=[]  NOutMax=[]  KbOutMin=[]  KbOutMax=[]  KtOutMin=[]  KtOutMax=[]  IntegratorOutMin=[]  IntegratorOutMax=[]  FilterOutMin=[]  FilterOutMax=[]  SumOutMin=[]  SumOutMax=[]  SumI1OutMin=[]  SumI1OutMax=[]  SumI2OutMin=[]  SumI2OutMax=[]  SumI3OutMin=[]  SumI3OutMax=[]  SumDOutMin=[]  SumDOutMax=[]  SaturationOutMin=[]  SaturationOutMax=[]  IntegratorContinuousStateAttributes=''  IntegratorStateMustResolveToSignalObject=off  IntegratorRTWStateStorageClass=Auto  FilterContinuousStateAttributes=''  FilterStateMustResolveToSignalObject=off  FilterRTWStateStorageClass=Auto  DifferentiatorICPrevScaledInput=0  DifferentiatorOutMin=[]  DifferentiatorOutMax=[]
  PID Controller7 : simulink/Continuous/PID Controller  Controller=PID  TimeDomain=Discrete-time  SampleTime=Tc  IntegratorMethod=Forward Euler  FilterMethod=Forward Euler  Form=Parallel  UseFilter=on  ControllerParametersSource=internal  P=0.015  I=0  D=0.25  N=3  InitialConditionSource=internal  InitialConditionForIntegrator=0  InitialConditionForFilter=0  ExternalReset=none  LimitOutput=off  UpperSaturationLimit=inf  LowerSaturationLimit=-inf  LinearizeAsGain=on  AntiWindupMode=none  Kb=1  TrackingMode=off  Kt=1  PParamMin=[]  PParamMax=[]  IParamMin=[]  IParamMax=[]  DParamMin=[]  DParamMax=[]  NParamMin=[]  NParamMax=[]  KbParamMin=[]  KbParamMax=[]  KtParamMin=[]  KtParamMax=[]  POutMin=[]  POutMax=[]  IOutMin=[]  IOutMax=[]  DOutMin=[]  DOutMax=[]  NOutMin=[]  NOutMax=[]  KbOutMin=[]  KbOutMax=[]  KtOutMin=[]  KtOutMax=[]  IntegratorOutMin=[]  IntegratorOutMax=[]  FilterOutMin=[]  FilterOutMax=[]  SumOutMin=[]  SumOutMax=[]  SumI1OutMin=[]  SumI1OutMax=[]  SumI2OutMin=[]  SumI2OutMax=[]  SumI3OutMin=[]  SumI3OutMax=[]  SumDOutMin=[]  SumDOutMax=[]  SaturationOutMin=[]  SaturationOutMax=[]  IntegratorContinuousStateAttributes=''  IntegratorStateMustResolveToSignalObject=off  IntegratorRTWStateStorageClass=Auto  FilterContinuousStateAttributes=''  FilterStateMustResolveToSignalObject=off  FilterRTWStateStorageClass=Auto  DifferentiatorICPrevScaledInput=0  DifferentiatorOutMin=[]  DifferentiatorOutMax=[]
  PID Controller8 : simulink/Continuous/PID Controller  Controller=PID  TimeDomain=Discrete-time  SampleTime=Tc  IntegratorMethod=Forward Euler  FilterMethod=Forward Euler  Form=Parallel  UseFilter=on  ControllerParametersSource=internal  P=-0.015  I=0  D=-0.25  N=3  InitialConditionSource=internal  InitialConditionForIntegrator=0  InitialConditionForFilter=0  ExternalReset=none  LimitOutput=off  UpperSaturationLimit=inf  LowerSaturationLimit=-inf  LinearizeAsGain=on  AntiWindupMode=none  Kb=1  TrackingMode=off  Kt=1  PParamMin=[]  PParamMax=[]  IParamMin=[]  IParamMax=[]  DParamMin=[]  DParamMax=[]  NParamMin=[]  NParamMax=[]  KbParamMin=[]  KbParamMax=[]  KtParamMin=[]  KtParamMax=[]  POutMin=[]  POutMax=[]  IOutMin=[]  IOutMax=[]  DOutMin=[]  DOutMax=[]  NOutMin=[]  NOutMax=[]  KbOutMin=[]  KbOutMax=[]  KtOutMin=[]  KtOutMax=[]  IntegratorOutMin=[]  IntegratorOutMax=[]  FilterOutMin=[]  FilterOutMax=[]  SumOutMin=[]  SumOutMax=[]  SumI1OutMin=[]  SumI1OutMax=[]  SumI2OutMin=[]  SumI2OutMax=[]  SumI3OutMin=[]  SumI3OutMax=[]  SumDOutMin=[]  SumDOutMax=[]  SaturationOutMin=[]  SaturationOutMax=[]  IntegratorContinuousStateAttributes=''  IntegratorStateMustResolveToSignalObject=off  IntegratorRTWStateStorageClass=Auto  FilterContinuousStateAttributes=''  FilterStateMustResolveToSignalObject=off  FilterRTWStateStorageClass=Auto  DifferentiatorICPrevScaledInput=0  DifferentiatorOutMin=[]  DifferentiatorOutMax=[]
  Pitch Controller Input : Subsystem  Variant=on
  Pitch Rate Controller Input : Subsystem  Variant=on
  Roll Controller Input : Subsystem  Variant=on
  Roll Rate Controller Input : Subsystem  Variant=on
  Saturation{,1..3} (4 alike) : Saturate  UpperLimit=20000  LowerLimit=-20000
  Scope{1..4,6,9,11..13} (9 alike) : Scope
  Sum{1..5,7,9..11} (9 alike) : Sum  Inputs=|+-
  To Workspace : ToWorkspace  VariableName=pitch_setpoint_model  SaveFormat=Structure With Time  SampleTime=-1
  To Workspace1 : ToWorkspace  VariableName=pitchrate_setpoint_model  SaveFormat=Structure With Time  SampleTime=Tq
  To Workspace10 : ToWorkspace  VariableName=yaw_value_model  SaveFormat=Structure With Time  SampleTime=Tc
  To Workspace11 : ToWorkspace  VariableName=y_position_model  SaveFormat=Structure With Time  SampleTime=Tc
  To Workspace12 : ToWorkspace  VariableName=z_position_model  SaveFormat=Structure With Time  SampleTime=Tc
  To Workspace2 : ToWorkspace  VariableName=x_command_model  SaveFormat=Structure With Time  SampleTime=Tq
  To Workspace3 : ToWorkspace  VariableName=roll_setpoint_model  SaveFormat=Structure With Time  SampleTime=Tc
  To Workspace4 : ToWorkspace  VariableName=rollrate_setpoint_model  SaveFormat=Structure With Time  SampleTime=Tq
  To Workspace5 : ToWorkspace  VariableName=y_command_model  SaveFormat=Structure With Time  SampleTime=Tq
  To Workspace6 : ToWorkspace  VariableName=z_command_model  SaveFormat=Structure With Time  SampleTime=Tq
  To Workspace7 : ToWorkspace  VariableName=yawrate_setpoint_model  SaveFormat=Structure With Time  SampleTime=Tc
  To Workspace8 : ToWorkspace  VariableName=yaw_command_model  SaveFormat=Structure With Time  SampleTime=Tq
  To Workspace9 : ToWorkspace  VariableName=x_position_model  SaveFormat=Structure With Time  SampleTime=Tc
  Yaw Controller Input : Subsystem  Variant=on
  Yaw Rate Controller Input : Subsystem  Variant=on
  height_controlled : Outport
  y_controlled : Outport  Port=2
  x_controlled : Outport  Port=3
  yaw_controlled : Outport  Port=4
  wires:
  pitch_rate/1 -> Scope6/1, Sum4/2
  z_setpoint/1 -> Sum7/1
  x_position/1 -> Scope4/1, To Workspace9/1, Sum5/2
  PID Controller5/1 -> Sum4/1, To Workspace1/1
  PID Controller8/1 -> Sum3/1, To Workspace/1
  pitch/1 -> Gain/1, Sum3/2
  Gain/1 -> Scope9/1
  PID Controller1/1 -> To Workspace8/1, Saturation/1
  PID Controller6/1 -> To Workspace2/1, Saturation1/1
  Latitude Controller Input/1(x_error) -> PID Controller8/1
  x_setpoint/1 -> Sum5/1
  roll_rate/1 -> Scope11/1, Sum10/2
  y_position/1 -> Scope12/1, To Workspace11/1, Sum11/2
  PID Controller2/1 -> Sum10/1, To Workspace4/1
  PID Controller7/1 -> Sum9/1, To Workspace3/1
  roll/1 -> Gain2/1, Sum9/2
  Gain2/1 -> Scope13/1
  y_setpoint/1 -> Sum11/1
  PID Controller17/1 -> To Workspace6/1, Saturation3/1
  yaw/1 -> Scope3/1, To Workspace10/1, Sum1/2
  yaw_setpoint/1 -> Sum1/1
  yaw_rate/1 -> Gain1/1, Sum2/2
  Gain1/1 -> Scope1/1
  PID Controller4/1 -> Sum2/1, To Workspace7/1
  z_position/1 -> To Workspace12/1, Scope2/1, Sum7/2
  Sum1/1 -> Yaw Controller Input/1(yaw_error_model)
  Yaw Controller Input/1(yaw_error) -> PID Controller4/1
  Sum2/1 -> Yaw Rate Controller Input/1(yawrate_error_model)
  Yaw Rate Controller Input/1(yawrate_error) -> PID Controller1/1
  Sum5/1 -> Latitude Controller Input/1(x_error_model)
  Sum3/1 -> Pitch Controller Input/1(pitch_error_model)
  Pitch Controller Input/1(pitch_error) -> PID Controller5/1
  Sum4/1 -> Pitch Rate Controller Input/1(pitchrate_error_model)
  Pitch Rate Controller Input/1(pitchrate_error) -> PID Controller6/1
  Sum11/1 -> Longitude Controller Input/1(y_error_model)
  Longitude Controller Input/1(y_error) -> PID Controller7/1
  Sum9/1 -> Roll Controller Input/1(roll_error_model)
  Roll Controller Input/1(roll_error) -> PID Controller2/1
  Sum10/1 -> Roll Rate Controller Input/1(rollrate_error_model)
  Altitude Controller Input/1(z_error) -> PID Controller17/1
  Sum7/1 -> Altitude Controller Input/1(z_error_model)
  Roll Rate Controller Input/1(rollrate_error) -> PID Controller3/1
  PID Controller3/1 -> To Workspace5/1, Saturation2/1
  Saturation3/1 -> height_controlled/1
  Saturation2/1 -> y_controlled/1
  Saturation1/1 -> x_controlled/1
  Saturation/1 -> yaw_controlled/1

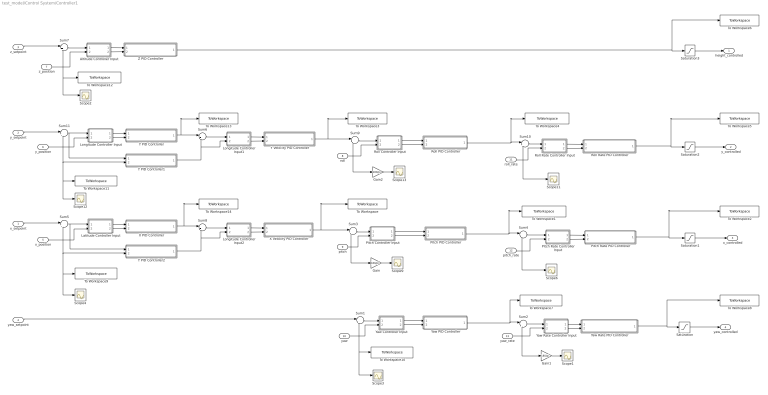
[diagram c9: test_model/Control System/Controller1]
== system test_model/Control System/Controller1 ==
  x_setpoint : Inport
  y_setpoint : Inport  Port=2
  z_setpoint : Inport  Port=3
  yaw_setpoint : Inport  Port=4
  x_position : Inport  Port=5
  y_position : Inport  Port=6
  z_position : Inport  Port=7
  roll : Inport  Port=8
  pitch : Inport  Port=9
  yaw : Inport  Port=10
  roll_rate : Inport  Port=11
  pitch_rate : Inport  Port=12
  yaw_rate : Inport  Port=13
  Altitude Controller Input : Subsystem  Variant=on
  Gain : Gain  Gain=180/pi
  Gain1 : Gain  Gain=180/pi
  Gain2 : Gain  Gain=180/pi
  Latitude Controller Input : Subsystem  Variant=on
  Longitude Controller Input : Subsystem  Variant=on
  Longitude Controller Input1 : Subsystem  Variant=on
  Longitude Controller Input2 : Subsystem  Variant=on
  Pitch Controller Input : Subsystem  Variant=on
  Pitch PID Controller : Subsystem
  Pitch Rate Controller Input : Subsystem  Variant=on
  Pitch Rate PID Controller : Subsystem
  Roll Controller Input : Subsystem  Variant=on
  Roll PID Controller : Subsystem
  Roll Rate Controller Input : Subsystem  Variant=on
  Roll Rate PID Controller : Subsystem
  Saturation{,1..3} (4 alike) : Saturate  UpperLimit=20000  LowerLimit=-20000
  Scope{1..4,6,9,11..13} (9 alike) : Scope
  Sum{1..11} (11 alike) : Sum  Inputs=|+-
  To Workspace : ToWorkspace  VariableName=pitch_setpoint_model  SaveFormat=Structure With Time  SampleTime=-1
  To Workspace1 : ToWorkspace  VariableName=pitchrate_setpoint_model  SaveFormat=Structure With Time  SampleTime=Tq
  To Workspace10 : ToWorkspace  VariableName=yaw_value_model  SaveFormat=Structure With Time  SampleTime=Tc
  To Workspace11 : ToWorkspace  VariableName=y_position_model  SaveFormat=Structure With Time  SampleTime=Tc
  To Workspace12 : ToWorkspace  VariableName=z_position_model  SaveFormat=Structure With Time  SampleTime=Tc
  To Workspace13 : ToWorkspace  VariableName=y_vel_setpoint_model  SaveFormat=Structure With Time  SampleTime=Tc
  To Workspace14 : ToWorkspace  VariableName=x_vel_setpoint_model  SaveFormat=Structure With Time  SampleTime=Tc
  To Workspace2 : ToWorkspace  VariableName=x_command_model  SaveFormat=Structure With Time  SampleTime=Tq
  To Workspace3 : ToWorkspace  VariableName=roll_setpoint_model  SaveFormat=Structure With Time  SampleTime=Tc
  To Workspace4 : ToWorkspace  VariableName=rollrate_setpoint_model  SaveFormat=Structure With Time  SampleTime=Tq
  To Workspace5 : ToWorkspace  VariableName=y_command_model  SaveFormat=Structure With Time  SampleTime=Tq
  To Workspace6 : ToWorkspace  VariableName=z_command_model  SaveFormat=Structure With Time  SampleTime=Tq
  To Workspace7 : ToWorkspace  VariableName=yawrate_setpoint_model  SaveFormat=Structure With Time  SampleTime=Tc
  To Workspace8 : ToWorkspace  VariableName=yaw_command_model  SaveFormat=Structure With Time  SampleTime=Tq
  To Workspace9 : ToWorkspace  VariableName=x_position_model  SaveFormat=Structure With Time  SampleTime=Tc
  X PID Controller : Subsystem
  X Velocity PID Controller : Subsystem
  Y PID Controller : Subsystem
  Y PID Controller1 : Subsystem
  Y PID Controller2 : Subsystem
  Y Velocity PID Controller : Subsystem
  Yaw Controller Input : Subsystem  Variant=on
  Yaw PID Controller : Subsystem
  Yaw Rate Controller Input : Subsystem  Variant=on
  Yaw Rate PID Controller : Subsystem
  Z PID Controller : Subsystem
  height_controlled : Outport
  y_controlled : Outport  Port=2
  x_controlled : Outport  Port=3
  yaw_controlled : Outport  Port=4
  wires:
  pitch_rate/1 -> Pitch Rate Controller Input/2(pitchrate_model), Scope6/1, Sum4/2
  z_setpoint/1 -> Sum7/1
  x_position/1 -> Sum5/2, Latitude Controller Input/2(x_position_model), Scope4/1, To Workspace9/1, Y PID Controller2/2(x_pos)
  Pitch PID Controller/1(pitchrate_setpoint) -> Sum4/1, To Workspace1/1
  pitch/1 -> Pitch Controller Input/2(pitch_angle_model), Gain/1, Sum3/2
  Gain/1 -> Scope9/1
  Yaw Rate PID Controller/1(yaw_motor_command) -> To Workspace8/1, Saturation/1
  Pitch Rate PID Controller/1(x_motor_command) -> Saturation1/1, To Workspace2/1
  x_setpoint/1 -> Sum5/1
  roll_rate/1 -> Roll Rate Controller Input/2(rollrate_model), Scope11/1, Sum10/2
  Roll PID Controller/1(rollrate_setpoint) -> Sum10/1, To Workspace4/1
  roll/1 -> Roll Controller Input/2(roll_angle_model), Gain2/1, Sum9/2
  Gain2/1 -> Scope13/1
  y_setpoint/1 -> Sum11/1
  Z PID Controller/1(z_motor_command) -> To Workspace6/1, Saturation3/1
  yaw/1 -> Yaw Controller Input/2(yaw_angle_model), Scope3/1, To Workspace10/1, Sum1/2
  yaw_setpoint/1 -> Sum1/1
  yaw_rate/1 -> Gain1/1, Yaw Rate Controller Input/2(yawrate_model), Sum2/2
  Gain1/1 -> Scope1/1
  Yaw PID Controller/1(yawrate_setpoint) -> Sum2/1, To Workspace7/1
  z_position/1 -> Altitude Controller Input/2(z_position_model), To Workspace12/1, Scope2/1, Sum7/2
  Sum1/1 -> Yaw Controller Input/1(yaw_error_model)
  Sum2/1 -> Yaw Rate Controller Input/1(yawrate_error_model)
  Sum5/1 -> Latitude Controller Input/1(x_error_model), Y PID Controller2/1(x_error)
  Sum3/1 -> Pitch Controller Input/1(pitch_error_model)
  Sum4/1 -> Pitch Rate Controller Input/1(pitchrate_error_model)
  Sum9/1 -> Roll Controller Input/1(roll_error_model)
  Sum10/1 -> Roll Rate Controller Input/1(rollrate_error_model)
  Sum7/1 -> Altitude Controller Input/1(z_error_model)
  Roll Rate PID Controller/1(y_motor_command) -> To Workspace5/1, Saturation2/1
  Saturation3/1 -> height_controlled/1
  Saturation2/1 -> y_controlled/1
  Saturation1/1 -> x_controlled/1
  Saturation/1 -> yaw_controlled/1
  Longitude Controller Input/2(y_position) -> Y PID Controller/2(y_pos)
  Longitude Controller Input/1(y_error) -> Y PID Controller/1(y_error)
  y_position/1 -> Longitude Controller Input/2(y_position_model), Y PID Controller1/2(y_pos), To Workspace11/1, Scope12/1, Sum11/2
  Latitude Controller Input/1(x_error) -> X PID Controller/1(x_error)
  Latitude Controller Input/2(x_position) -> X PID Controller/2(x_pos)
  Yaw Controller Input/1(yaw_error) -> Yaw PID Controller/1(yaw_error)
  Yaw Controller Input/2(yaw_angle) -> Yaw PID Controller/2(yaw_angle)
  Altitude Controller Input/1(z_error) -> Z PID Controller/1(z_error)
  Altitude Controller Input/2(z_position) -> Z PID Controller/2(z_pos)
  Pitch Controller Input/1(pitch_error) -> Pitch PID Controller/1(pitch_error)
  Pitch Controller Input/2(pitch_angle) -> Pitch PID Controller/2(pitch_angle)
  Yaw Rate Controller Input/1(yawrate_error) -> Yaw Rate PID Controller/1(yawrate_error)
  Yaw Rate Controller Input/2(yawrate) -> Yaw Rate PID Controller/2(yawrate)
  Pitch Rate Controller Input/1(pitchrate_error) -> Pitch Rate PID Controller/1(pitchrate_error)
  Pitch Rate Controller Input/2(pitchrate) -> Pitch Rate PID Controller/2(pitchrate)
  Roll Controller Input/1(roll_error) -> Roll PID Controller/1(roll_error)
  Roll Controller Input/2(roll_angle) -> Roll PID Controller/2(roll_angle)
  Roll Rate Controller Input/1(rollrate_error) -> Roll Rate PID Controller/1(rollrate_error)
  Roll Rate Controller Input/2(rollrate) -> Roll Rate PID Controller/2(rollrate)
  Sum11/1 -> Longitude Controller Input/1(y_error_model), Y PID Controller1/1(y_error)
  Y PID Controller/1(roll_setpoint) -> To Workspace13/1, Sum6/1
  Y PID Controller1/1(y_vel_setpoint) -> Longitude Controller Input1/2(y_vel_model), Sum6/2
  Sum6/1 -> Longitude Controller Input1/1(y_vel_error_model)
  Longitude Controller Input1/1(y_vel_error) -> Y Velocity PID Controller/1(y_error)
  Longitude Controller Input1/2(y_vel) -> Y Velocity PID Controller/2(y_pos)
  Y Velocity PID Controller/1(roll_setpoint) -> To Workspace3/1, Sum9/1
  X PID Controller/1(pitch_setpoint) -> To Workspace14/1, Sum8/1
  Y PID Controller2/1(x_vel_setpoint) -> Longitude Controller Input2/2(x_vel_model), Sum8/2
  Sum8/1 -> Longitude Controller Input2/1(x_vel_error_model)
  Longitude Controller Input2/1(x_vel_error) -> X Velocity PID Controller/1(x_vel_error)
  Longitude Controller Input2/2(x_vel) -> X Velocity PID Controller/2(x_vel)
  X Velocity PID Controller/1(pitch_setpoint) -> To Workspace/1, Sum3/1

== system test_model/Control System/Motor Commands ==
  note: 1) Add Subsystem or Model blocks as valid variant choices. 2) You cannot connect blocks at this level. At simulation, connectivity is automatically determined, based on the active variant and port name matching.
  z_command_model : Inport
  Feedback : Subsystem  VariantControl=logAnalysisToggle==0
  Motor Command : Subsystem  VariantControl=logAnalysisToggle==1
  z_command : Outport

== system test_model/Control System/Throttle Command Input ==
  note: 1) Add Subsystem or Model blocks as valid variant choices. 2) You cannot connect blocks at this level. At simulation, connectivity is automatically determined, based on the active variant and port name matching.
  z_command_model : Inport
  Feedback : Subsystem  VariantControl=logAnalysisToggle==0
  Throttle Command : Subsystem  VariantControl=logAnalysisToggle==1
  z_command : Outport

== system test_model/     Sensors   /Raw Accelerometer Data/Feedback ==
  raw_accel_model : Inport
  raw_accel : Outport
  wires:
  raw_accel_model/1 -> raw_accel/1

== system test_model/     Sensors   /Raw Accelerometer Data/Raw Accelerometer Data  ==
  From Workspace5 : FromWorkspace  VariableName=raw_accel_data  SampleTime=Tq
  raw_accel : Outport
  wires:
  From Workspace5/1 -> raw_accel/1

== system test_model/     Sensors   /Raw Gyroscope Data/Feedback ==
  raw_gyro_model : Inport
  raw_gyro : Outport
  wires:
  raw_gyro_model/1 -> raw_gyro/1
